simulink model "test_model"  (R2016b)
settings: Solver=VariableStepAuto  StartTime=0.0  StopTime=runtime  RelTol=1e-3
InitFcn:
  | clear mex
  | delete test_model_sfun.mexw64
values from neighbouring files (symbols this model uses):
  delta_T = 4 * [ 0,  0,  2.351e-4 ]    [modelParameters.m]
  Delta_T = cell(1,4)    [modelParameters.m]
  F_D = 1*randn(3,1)    [modelParameters.m]
  g = 9.81    [modelParameters.m]    (also in analyzeIMU_data.m = 9.8; getMomentOfInertia.m = 9.80665)
  Gamma_H = cell(1,4)    [modelParameters.m]
  have_motor_transient = 1    [modelParameters.m]
  height_controlled_o = (((Rm*If        + (((omega0_o * 2 * Rm * Kv * Kq      * Kd + 1)^2) - 1)/(4* Rm*Kv^2*Kq      * Kd))/Vb)*(Pmax - Pmin) + Pmin)    [modelParameters.m]
  i_0 = cell(1,4)    [modelParameters.m]
  If = 0.3836    [modelParameters.m]    (also in thrustDragConstantCalculations.m = [If0; If1; If2; If3]; Kd_error.m = I_0 * sign(rotor_speed_0) + I_1 * rotor_speed_0 + I_2 * roto)
  J = diag([ 0.0130 0.0140 0.0285 ])    [modelParameters.m]    (also in J_calc_bifilar.m = (16*pi^2*L./(m*g.*D.^2))\(t./n).^2)
  J_L = m_L/12*diag([y_L^2+z_L^2,x_L^2+z_L^2,x_L^2+y_L^2])    [modelParameters.m]
  J_r = cell(1,4)    [modelParameters.m]
  Jreq = 4.2012e-05    [modelParameters.m]
  Jxx = 0.0130    (= 0.013)    [modelParameters.m]
  Jyy = 0.0140    (= 0.014)    [modelParameters.m]
  Jzz = 0.0285    [modelParameters.m]
  K_d = cell(1,4)    [modelParameters.m]
  K_E = cell(1,4)    [modelParameters.m]
  K_H = cell(1,4)    [modelParameters.m]
  K_Q = cell(1,4)    [modelParameters.m]
  K_T = cell(1,4)    [modelParameters.m]
  K_V = cell(1,4)    [modelParameters.m]
  Kd = 1.4852e-07    [modelParameters.m]    (also in calcDragConstant.m = ((A'*A)^-1)*A'*b; thrustDragConstantCalculations.m = calcDragConstant(data, Pmin, Pmax, Rm, Kv, Kq, If); Kd_error.m = 1.0317e-07)
  Kh = 3.4574e-04    (= 0.00034574)    [modelParameters.m]
  Ki_mahony = 0.001    [modelParameters.m]
  Kp_mahony = 0.4    [modelParameters.m]
  Kq = 96.3422    [modelParameters.m]    (also in thrustDragConstantCalculations.m; Kd_error.m)
  Kt = 1.2007e-05    [modelParameters.m]    (also in calcThrustConstant.m = ((A'*A)^(-1))*(A'*T); thrustDragConstantCalculations.m = calcThrustConstant(data))
  Kv = 96.3422    [modelParameters.m]    (also in thrustDragConstantCalculations.m; Kd_error.m)
  m = 1.216    [modelParameters.m]
  m_L = 0    [modelParameters.m]
  omega0_o = sqrt((m*g)/(4*Kt))    [modelParameters.m]
  omega1_o = sqrt((m*g)/(4*Kt))    [modelParameters.m]
  omega2_o = sqrt((m*g)/(4*Kt))    [modelParameters.m]
  omega3_o = sqrt((m*g)/(4*Kt))    [modelParameters.m]
  omega_0 = cell(1,4)    [modelParameters.m]
  p0 = 0    [modelParameters.m]
  p_0 = cell(1,4)    [modelParameters.m]
  p_max = cell(1,4)    [modelParameters.m]
  phi0 = 0    [modelParameters.m]
  pitch_o = 0    [modelParameters.m]
  pitchrate_o = 0    [modelParameters.m]
  Pmax = 1    [modelParameters.m]    (also in thrustDragConstantCalculations.m = 200000; Kd_error.m = 200000)
  Pmin = 0    [modelParameters.m]    (also in thrustDragConstantCalculations.m = 100000; Kd_error.m = 100000)
  psi0 = 0    [modelParameters.m]
  q0 = 0    [modelParameters.m]
  Q_D = 0.05*randn(3,1)    [modelParameters.m]
  r0 = 0    [modelParameters.m]
  R_m = cell(1,4)    [modelParameters.m]
  r_oc = [ 0 ; 0 ; 0 ]    [modelParameters.m]
  r_oL = [0; 0; 0]    [modelParameters.m]
  rhx = 0.16    [modelParameters.m]
  rhy = 0.16    [modelParameters.m]
  rhz = 0.03    [modelParameters.m]
  Rm = 0.235    [modelParameters.m]    (also in thrustDragConstantCalculations.m = 0.2308; Kd_error.m = 0.2308)
  roll_o = 0    [modelParameters.m]
  rollrate_o = 0    [modelParameters.m]
  Tc = 0.04    [modelParameters.m]
  theta0 = 0    [modelParameters.m]
  Tq = 0.005    [modelParameters.m]
  u0 = 0    [modelParameters.m]
  v0 = 0    [modelParameters.m]
  Vb = 12.3    [modelParameters.m]    (also in calcDragConstant.m = [data.(6); data.(6); data.(6); data.(6)]; Kd_error.m = data.(6))
  w0 = 0    [modelParameters.m]
  x0 = 0    [modelParameters.m]
  x_controlled_o = 0    [modelParameters.m]
  x_o = 0    [modelParameters.m]
  x_vel_o = 0    [modelParameters.m]
  y0 = 0    [modelParameters.m]
  y_controlled_o = 0    [modelParameters.m]
  y_o = 0    [modelParameters.m]
  y_vel_o = 0    [modelParameters.m]
  yaw_controlled_o = 0    [modelParameters.m]
  yaw_o = 0    [modelParameters.m]
  yawrate_o = 0    [modelParameters.m]
  z0 = 0    [modelParameters.m]
  z_o = 0    [modelParameters.m]
  z_vel_o = 0    [modelParameters.m]
undefined symbols (not defined in the file or in its folder): Gamma_Omega, Gamma_T, Ki, Kp, r_h, slope, start, Ts, X0
libraries: simulink x32, Derivative x26, dsparch4 x6, vrlib x4
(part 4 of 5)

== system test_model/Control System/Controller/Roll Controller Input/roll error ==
  From Workspace1 : FromWorkspace  VariableName=roll_angle  SampleTime=Tq  Interpolate=off  OutputAfterFinalValue=Holding final value
  From Workspace4 : FromWorkspace  VariableName=roll_error  SampleTime=Tq  Interpolate=off  OutputAfterFinalValue=Holding final value
  roll_error : Outport
  roll_angle : Outport  Port=2
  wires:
  From Workspace4/1 -> roll_error/1
  From Workspace1/1 -> roll_angle/1

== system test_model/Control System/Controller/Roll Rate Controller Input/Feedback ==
  rollrate_error_model : Inport
  rollrate_model : Inport  Port=2
  rollrate_error : Outport
  rollrate : Outport  Port=2
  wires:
  rollrate_error_model/1 -> rollrate_error/1
  rollrate_model/1 -> rollrate/1

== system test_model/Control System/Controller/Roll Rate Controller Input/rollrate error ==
  From Workspace1 : FromWorkspace  VariableName=rollrate  SampleTime=Tq  Interpolate=off  OutputAfterFinalValue=Holding final value
  From Workspace5 : FromWorkspace  VariableName=rollrate_error  SampleTime=Tq  Interpolate=off  OutputAfterFinalValue=Holding final value
  rollrate_error : Outport
  rollrate : Outport  Port=2
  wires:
  From Workspace5/1 -> rollrate_error/1
  From Workspace1/1 -> rollrate/1

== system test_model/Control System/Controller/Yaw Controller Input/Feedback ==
  yaw_error_model : Inport
  yaw_angle_model : Inport  Port=2
  yaw_error : Outport
  yaw_angle : Outport  Port=2
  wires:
  yaw_error_model/1 -> yaw_error/1
  yaw_angle_model/1 -> yaw_angle/1

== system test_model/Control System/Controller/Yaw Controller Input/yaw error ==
  From Workspace1 : FromWorkspace  VariableName=yaw_angle  SampleTime=Tc  Interpolate=off  OutputAfterFinalValue=Holding final value
  From Workspace7 : FromWorkspace  VariableName=yaw_error  SampleTime=Tc  Interpolate=off  OutputAfterFinalValue=Holding final value
  yaw_error : Outport
  yaw_angle : Outport  Port=2
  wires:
  From Workspace7/1 -> yaw_error/1
  From Workspace1/1 -> yaw_angle/1

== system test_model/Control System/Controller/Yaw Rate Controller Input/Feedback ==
  yawrate_error_model : Inport
  yawrate_model : Inport  Port=2
  yawrate_error : Outport
  yawrate : Outport  Port=2
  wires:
  yawrate_error_model/1 -> yawrate_error/1
  yawrate_model/1 -> yawrate/1

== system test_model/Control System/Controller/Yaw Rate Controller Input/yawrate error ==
  From Workspace1 : FromWorkspace  VariableName=yawrate  SampleTime=Tq  Interpolate=off  OutputAfterFinalValue=Holding final value
  From Workspace8 : FromWorkspace  VariableName=yawrate_error  SampleTime=Tq  Interpolate=off  OutputAfterFinalValue=Holding final value
  yawrate_error : Outport
  yawrate : Outport  Port=2
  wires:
  From Workspace8/1 -> yawrate_error/1
  From Workspace1/1 -> yawrate/1

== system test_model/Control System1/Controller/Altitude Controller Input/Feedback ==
  z_error_model : Inport
  z_position_model : Inport  Port=2
  z_error : Outport
  z_position : Outport  Port=2
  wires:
  z_error_model/1 -> z_error/1
  z_position_model/1 -> z_position/1

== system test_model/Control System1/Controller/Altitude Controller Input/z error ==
  From Workspace1 : FromWorkspace  VariableName=z_position  SampleTime=Tc  Interpolate=off  OutputAfterFinalValue=Holding final value
  From Workspace6 : FromWorkspace  VariableName=z_error  SampleTime=Tc  Interpolate=off  OutputAfterFinalValue=Holding final value
  z_error : Outport
  z_position : Outport  Port=2
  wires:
  From Workspace6/1 -> z_error/1
  From Workspace1/1 -> z_position/1

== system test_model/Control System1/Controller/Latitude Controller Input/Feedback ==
  x_error_model : Inport
  x_position_model : Inport  Port=2
  x_error : Outport
  x_position : Outport  Port=2
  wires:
  x_error_model/1 -> x_error/1
  x_position_model/1 -> x_position/1

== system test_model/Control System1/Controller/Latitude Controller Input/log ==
  From Workspace : FromWorkspace  VariableName=x_error  SampleTime=Tc  Interpolate=off  OutputAfterFinalValue=Holding final value
  From Workspace1 : FromWorkspace  VariableName=x_position  SampleTime=Tc  Interpolate=off  OutputAfterFinalValue=Holding final value
  x_error : Outport
  x_position : Outport  Port=2
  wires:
  From Workspace/1 -> x_error/1
  From Workspace1/1 -> x_position/1

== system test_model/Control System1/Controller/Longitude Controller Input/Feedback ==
  y_error_model : Inport
  y_position_model : Inport  Port=2
  y_error : Outport
  y_position : Outport  Port=2
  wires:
  y_error_model/1 -> y_error/1
  y_position_model/1 -> y_position/1

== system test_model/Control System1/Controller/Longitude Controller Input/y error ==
  From Workspace1 : FromWorkspace  VariableName=y_position  SampleTime=Tc  Interpolate=off  OutputAfterFinalValue=Holding final value
  From Workspace3 : FromWorkspace  VariableName=y_error  SampleTime=Tc  Interpolate=off  OutputAfterFinalValue=Holding final value
  y_error : Outport
  y_position : Outport  Port=2
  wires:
  From Workspace3/1 -> y_error/1
  From Workspace1/1 -> y_position/1

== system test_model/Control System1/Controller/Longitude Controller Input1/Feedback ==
  y_vel_error_model : Inport
  y_vel_model : Inport  Port=2
  y_vel_error : Outport
  y_vel : Outport  Port=2
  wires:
  y_vel_error_model/1 -> y_vel_error/1
  y_vel_model/1 -> y_vel/1

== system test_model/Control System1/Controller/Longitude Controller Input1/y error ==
  From Workspace1 : FromWorkspace  VariableName=y_vel  SampleTime=Tc  Interpolate=off  OutputAfterFinalValue=Holding final value
  From Workspace3 : FromWorkspace  VariableName=y_vel_error  SampleTime=Tc  Interpolate=off  OutputAfterFinalValue=Holding final value
  y_vel_error : Outport
  y_vel : Outport  Port=2
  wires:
  From Workspace3/1 -> y_vel_error/1
  From Workspace1/1 -> y_vel/1

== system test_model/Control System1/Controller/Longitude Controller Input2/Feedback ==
  x_vel_error_model : Inport
  x_vel_model : Inport  Port=2
  x_vel_error : Outport
  x_vel : Outport  Port=2
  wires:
  x_vel_error_model/1 -> x_vel_error/1
  x_vel_model/1 -> x_vel/1

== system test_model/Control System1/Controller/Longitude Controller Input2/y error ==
  From Workspace1 : FromWorkspace  VariableName=x_vel  SampleTime=Tc  Interpolate=off  OutputAfterFinalValue=Holding final value
  From Workspace3 : FromWorkspace  VariableName=x_vel_error  SampleTime=Tc  Interpolate=off  OutputAfterFinalValue=Holding final value
  x_vel_error : Outport
  x_vel : Outport  Port=2
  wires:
  From Workspace3/1 -> x_vel_error/1
  From Workspace1/1 -> x_vel/1

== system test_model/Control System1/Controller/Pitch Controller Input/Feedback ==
  pitch_error_model : Inport
  pitch_angle_model : Inport  Port=2
  pitch_error : Outport
  pitch_angle : Outport  Port=2
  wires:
  pitch_error_model/1 -> pitch_error/1
  pitch_angle_model/1 -> pitch_angle/1

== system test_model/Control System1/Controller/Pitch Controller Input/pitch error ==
  From Workspace : FromWorkspace  VariableName=pitch_error  SampleTime=Tq  Interpolate=off  OutputAfterFinalValue=Holding final value
  From Workspace1 : FromWorkspace  VariableName=pitch_angle  SampleTime=Tq  Interpolate=off  OutputAfterFinalValue=Holding final value
  pitch_error : Outport
  pitch_angle : Outport  Port=2
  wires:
  From Workspace/1 -> pitch_error/1
  From Workspace1/1 -> pitch_angle/1

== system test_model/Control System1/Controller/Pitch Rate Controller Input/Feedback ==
  pitchrate_error_model : Inport
  pitchrate_model : Inport  Port=2
  pitchrate_error : Outport
  pitchrate : Outport  Port=2
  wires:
  pitchrate_error_model/1 -> pitchrate_error/1
  pitchrate_model/1 -> pitchrate/1

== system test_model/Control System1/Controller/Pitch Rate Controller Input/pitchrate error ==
  From Workspace1 : FromWorkspace  VariableName=pitchrate  SampleTime=Tq  Interpolate=off  OutputAfterFinalValue=Holding final value
  From Workspace2 : FromWorkspace  VariableName=pitchrate_error  SampleTime=Tq  Interpolate=off  OutputAfterFinalValue=Holding final value
  pitchrate_error : Outport
  pitchrate : Outport  Port=2
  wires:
  From Workspace2/1 -> pitchrate_error/1
  From Workspace1/1 -> pitchrate/1

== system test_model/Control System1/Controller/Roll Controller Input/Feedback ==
  roll_error_model : Inport
  roll_angle_model : Inport  Port=2
  roll_error : Outport
  roll_angle : Outport  Port=2
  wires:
  roll_error_model/1 -> roll_error/1
  roll_angle_model/1 -> roll_angle/1

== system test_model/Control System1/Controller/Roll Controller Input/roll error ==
  From Workspace1 : FromWorkspace  VariableName=roll_angle  SampleTime=Tq  Interpolate=off  OutputAfterFinalValue=Holding final value
  From Workspace4 : FromWorkspace  VariableName=roll_error  SampleTime=Tq  Interpolate=off  OutputAfterFinalValue=Holding final value
  roll_error : Outport
  roll_angle : Outport  Port=2
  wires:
  From Workspace4/1 -> roll_error/1
  From Workspace1/1 -> roll_angle/1

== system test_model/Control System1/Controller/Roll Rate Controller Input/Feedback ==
  rollrate_error_model : Inport
  rollrate_model : Inport  Port=2
  rollrate_error : Outport
  rollrate : Outport  Port=2
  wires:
  rollrate_error_model/1 -> rollrate_error/1
  rollrate_model/1 -> rollrate/1

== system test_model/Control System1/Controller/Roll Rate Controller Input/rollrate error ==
  From Workspace1 : FromWorkspace  VariableName=rollrate  SampleTime=Tq  Interpolate=off  OutputAfterFinalValue=Holding final value
  From Workspace5 : FromWorkspace  VariableName=rollrate_error  SampleTime=Tq  Interpolate=off  OutputAfterFinalValue=Holding final value
  rollrate_error : Outport
  rollrate : Outport  Port=2
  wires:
  From Workspace5/1 -> rollrate_error/1
  From Workspace1/1 -> rollrate/1

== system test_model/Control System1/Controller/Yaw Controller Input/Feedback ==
  yaw_error_model : Inport
  yaw_angle_model : Inport  Port=2
  yaw_error : Outport
  yaw_angle : Outport  Port=2
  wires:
  yaw_error_model/1 -> yaw_error/1
  yaw_angle_model/1 -> yaw_angle/1

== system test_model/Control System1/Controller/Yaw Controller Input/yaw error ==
  From Workspace1 : FromWorkspace  VariableName=yaw_angle  SampleTime=Tc  Interpolate=off  OutputAfterFinalValue=Holding final value
  From Workspace7 : FromWorkspace  VariableName=yaw_error  SampleTime=Tc  Interpolate=off  OutputAfterFinalValue=Holding final value
  yaw_error : Outport
  yaw_angle : Outport  Port=2
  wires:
  From Workspace7/1 -> yaw_error/1
  From Workspace1/1 -> yaw_angle/1

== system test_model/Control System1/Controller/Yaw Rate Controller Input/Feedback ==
  yawrate_error_model : Inport
  yawrate_model : Inport  Port=2
  yawrate_error : Outport
  yawrate : Outport  Port=2
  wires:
  yawrate_error_model/1 -> yawrate_error/1
  yawrate_model/1 -> yawrate/1

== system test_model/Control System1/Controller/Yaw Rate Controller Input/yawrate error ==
  From Workspace1 : FromWorkspace  VariableName=yawrate  SampleTime=Tq  Interpolate=off  OutputAfterFinalValue=Holding final value
  From Workspace8 : FromWorkspace  VariableName=yawrate_error  SampleTime=Tq  Interpolate=off  OutputAfterFinalValue=Holding final value
  yawrate_error : Outport
  yawrate : Outport  Port=2
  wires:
  From Workspace8/1 -> yawrate_error/1
  From Workspace1/1 -> yawrate/1

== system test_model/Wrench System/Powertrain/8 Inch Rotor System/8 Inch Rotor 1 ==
  alpha : Inport
  omega : Inport  Port=2
  v : Inport  Port=3
  Omega : Inport  Port=4
  8 Inch Rotor : MATLAB Function
  Delta_T : Constant  Value=Delta_T
  Gamma_H : Constant  Value=Gamma_H
  Gamma_Omega : Constant  Value=Gamma_Omega
  Gamma_T : Constant  Value=Gamma_T
  J_r : Constant  Value=J_r
  K_H : Constant  Value=K_H
  K_T : Constant  Value=K_T
  K_d : Constant  Value=K_d
  Scope : Scope
  r_h : Constant  Value=r_h
  F : Outport
  Q : Outport  Port=2
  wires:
  8 Inch Rotor/2(Q) -> Q/1
  8 Inch Rotor/1(F) -> Scope/1, F/1
  Omega/1 -> 8 Inch Rotor/4(Omega)
  v/1 -> 8 Inch Rotor/3(v)
  K_T/1 -> 8 Inch Rotor/5(K_T)
  Gamma_Omega/1 -> 8 Inch Rotor/12(Gamma_Omega)
  Gamma_H/1 -> 8 Inch Rotor/11(Gamma_H)
  Gamma_T/1 -> 8 Inch Rotor/10(Gamma_T)
  Delta_T/1 -> 8 Inch Rotor/9(Delta_T)
  r_h/1 -> 8 Inch Rotor/8(r_h)
  K_d/1 -> 8 Inch Rotor/7(K_d)
  K_H/1 -> 8 Inch Rotor/6(K_H)
  omega/1 -> 8 Inch Rotor/1(omega)
  alpha/1 -> 8 Inch Rotor/2(alpha)
  J_r/1 -> 8 Inch Rotor/13(J_r)

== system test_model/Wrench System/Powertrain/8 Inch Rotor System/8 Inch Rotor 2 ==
  alpha : Inport
  omega : Inport  Port=2
  v : Inport  Port=3
  Omega : Inport  Port=4
  8 Inch Rotor : MATLAB Function
  Delta_T : Constant  Value=Delta_T
  Gamma_H : Constant  Value=Gamma_H
  Gamma_Omega : Constant  Value=Gamma_Omega
  Gamma_T : Constant  Value=Gamma_T
  J_r : Constant  Value=J_r
  K_H : Constant  Value=K_H
  K_T : Constant  Value=K_T
  K_d : Constant  Value=K_d
  r_h : Constant  Value=r_h
  F : Outport
  Q : Outport  Port=2
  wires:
  8 Inch Rotor/2(Q) -> Q/1
  8 Inch Rotor/1(F) -> F/1
  Omega/1 -> 8 Inch Rotor/4(Omega)
  v/1 -> 8 Inch Rotor/3(v)
  K_T/1 -> 8 Inch Rotor/5(K_T)
  Gamma_Omega/1 -> 8 Inch Rotor/12(Gamma_Omega)
  Gamma_H/1 -> 8 Inch Rotor/11(Gamma_H)
  Gamma_T/1 -> 8 Inch Rotor/10(Gamma_T)
  Delta_T/1 -> 8 Inch Rotor/9(Delta_T)
  r_h/1 -> 8 Inch Rotor/8(r_h)
  K_d/1 -> 8 Inch Rotor/7(K_d)
  K_H/1 -> 8 Inch Rotor/6(K_H)
  omega/1 -> 8 Inch Rotor/1(omega)
  alpha/1 -> 8 Inch Rotor/2(alpha)
  J_r/1 -> 8 Inch Rotor/13(J_r)

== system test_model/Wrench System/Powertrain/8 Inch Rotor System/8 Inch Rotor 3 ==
  alpha : Inport
  omega : Inport  Port=2
  v : Inport  Port=3
  Omega : Inport  Port=4
  8 Inch Rotor : MATLAB Function
  Delta_T : Constant  Value=Delta_T
  Gamma_H : Constant  Value=Gamma_H
  Gamma_Omega : Constant  Value=Gamma_Omega
  Gamma_T : Constant  Value=Gamma_T
  J_r : Constant  Value=J_r
  K_H : Constant  Value=K_H
  K_T : Constant  Value=K_T
  K_d : Constant  Value=K_d
  r_h : Constant  Value=r_h
  F : Outport
  Q : Outport  Port=2
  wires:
  8 Inch Rotor/2(Q) -> Q/1
  8 Inch Rotor/1(F) -> F/1
  Omega/1 -> 8 Inch Rotor/4(Omega)
  v/1 -> 8 Inch Rotor/3(v)
  K_T/1 -> 8 Inch Rotor/5(K_T)
  Gamma_Omega/1 -> 8 Inch Rotor/12(Gamma_Omega)
  Gamma_H/1 -> 8 Inch Rotor/11(Gamma_H)
  Gamma_T/1 -> 8 Inch Rotor/10(Gamma_T)
  Delta_T/1 -> 8 Inch Rotor/9(Delta_T)
  r_h/1 -> 8 Inch Rotor/8(r_h)
  K_d/1 -> 8 Inch Rotor/7(K_d)
  K_H/1 -> 8 Inch Rotor/6(K_H)
  omega/1 -> 8 Inch Rotor/1(omega)
  alpha/1 -> 8 Inch Rotor/2(alpha)
  J_r/1 -> 8 Inch Rotor/13(J_r)

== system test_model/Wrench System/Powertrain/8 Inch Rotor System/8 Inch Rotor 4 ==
  alpha : Inport
  omega : Inport  Port=2
  v : Inport  Port=3
  Omega : Inport  Port=4
  8 Inch Rotor : MATLAB Function
  Delta_T : Constant  Value=Delta_T
  Gamma_H : Constant  Value=Gamma_H
  Gamma_Omega : Constant  Value=Gamma_Omega
  Gamma_T : Constant  Value=Gamma_T
  J_r : Constant  Value=J_r
  K_H : Constant  Value=K_H
  K_T : Constant  Value=K_T
  K_d : Constant  Value=K_d
  r_h : Constant  Value=r_h
  F : Outport
  Q : Outport  Port=2
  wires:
  8 Inch Rotor/2(Q) -> Q/1
  8 Inch Rotor/1(F) -> F/1
  Omega/1 -> 8 Inch Rotor/4(Omega)
  v/1 -> 8 Inch Rotor/3(v)
  K_T/1 -> 8 Inch Rotor/5(K_T)
  Gamma_Omega/1 -> 8 Inch Rotor/12(Gamma_Omega)
  Gamma_H/1 -> 8 Inch Rotor/11(Gamma_H)
  Gamma_T/1 -> 8 Inch Rotor/10(Gamma_T)
  Delta_T/1 -> 8 Inch Rotor/9(Delta_T)
  r_h/1 -> 8 Inch Rotor/8(r_h)
  K_d/1 -> 8 Inch Rotor/7(K_d)
  K_H/1 -> 8 Inch Rotor/6(K_H)
  omega/1 -> 8 Inch Rotor/1(omega)
  alpha/1 -> 8 Inch Rotor/2(alpha)
  J_r/1 -> 8 Inch Rotor/13(J_r)

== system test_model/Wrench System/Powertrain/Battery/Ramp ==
  Clock : Clock
  Constant : Constant  DisableCoverage=on  Value=start  OutDataTypeStr=Inherit: Inherit via back propagation
  Constant1 : Constant  DisableCoverage=on  Value=X0  OutDataTypeStr=Inherit: Inherit via back propagation
  Output : Sum  Inputs=|++
  Product : Product  DisableCoverage=on
  Step : Step  DisableCoverage=on  Time=start  After=slope  SampleTime=0
  Sum : Sum  DisableCoverage=on  Inputs=|+-
  Out1 : Outport
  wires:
  Clock/1 -> Sum/1
  Constant/1 -> Sum/2
  Sum/1 -> Product/2
  Output/1 -> Out1/1
  Constant1/1 -> Output/2
  Product/1 -> Output/1
  Step/1 -> Product/1

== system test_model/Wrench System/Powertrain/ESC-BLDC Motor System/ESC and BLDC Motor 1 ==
  p : Inport
  V_b : Inport  Port=2
  "BLDC Motor " : MATLAB Function  TreatAsAtomicUnit=on
  BLDC Motor (no transient) : MATLAB Function  TreatAsAtomicUnit=on
  "ESC " : MATLAB Function  TreatAsAtomicUnit=on
  Integrator : Integrator  InitialCondition=omega_0  ContinuousStateAttributes='omega'
  J_r : Constant  Value=J_r
  K_E : Constant  Value=K_E
  K_Q : Constant  Value=K_Q
  K_V : Constant  Value=K_V
  K_d : Constant  Value=K_d
  R_m : Constant  Value=R_m
  alpha_switch : Switch  Criteria=u2 ~= 0
  i_0 : Constant  Value=i_0
  motor_transient_choice : Constant  Value=have_motor_transient
  omega_switch : Switch  Criteria=u2 ~= 0
  p_0 : Constant  Value=p_0
  p_max : Constant  Value=p_max
  alpha : Outport
  omega : Outport  Port=2
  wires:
  motor_transient_choice/1 -> omega_switch/2, alpha_switch/2
  omega_switch/1 -> omega/1
  alpha_switch/1 -> alpha/1
  BLDC Motor (no transient)/2(omega) -> omega_switch/3
  BLDC Motor (no transient)/1(alpha) -> alpha_switch/3
  Integrator/1 -> omega_switch/1, "BLDC Motor "/2(omega)
  "ESC "/1(V) -> BLDC Motor (no transient)/1(V), "BLDC Motor "/1(V)
  p/1 -> "ESC "/1(p)
  V_b/1 -> "ESC "/2(V_b)
  K_E/1 -> "ESC "/3(K_E)
  p_0/1 -> "ESC "/4(p_0)
  p_max/1 -> "ESC "/5(p_max)
  J_r/1 -> "BLDC Motor "/8(J_r)
  R_m/1 -> BLDC Motor (no transient)/2(R_m), "BLDC Motor "/3(R_m)
  "BLDC Motor "/1(alpha) -> alpha_switch/1, Integrator/1
  K_Q/1 -> BLDC Motor (no transient)/3(K_Q), "BLDC Motor "/4(K_Q)
  K_V/1 -> BLDC Motor (no transient)/4(K_V), "BLDC Motor "/5(K_V)
  i_0/1 -> BLDC Motor (no transient)/5(i_0), "BLDC Motor "/6(i_0)
  K_d/1 -> BLDC Motor (no transient)/6(K_d), "BLDC Motor "/7(K_d)

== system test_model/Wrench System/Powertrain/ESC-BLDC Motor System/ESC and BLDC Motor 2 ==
  p : Inport
  V_b : Inport  Port=2
  "BLDC Motor " : MATLAB Function  TreatAsAtomicUnit=on
  BLDC Motor (no transient) : MATLAB Function  TreatAsAtomicUnit=on
  "ESC " : MATLAB Function  TreatAsAtomicUnit=on
  Integrator : Integrator  InitialCondition=omega_0  ContinuousStateAttributes='omega'
  J_r : Constant  Value=J_r
  K_E : Constant  Value=K_E
  K_Q : Constant  Value=K_Q
  K_V : Constant  Value=K_V
  K_d : Constant  Value=K_d
  R_m : Constant  Value=R_m
  alpha_switch : Switch  Criteria=u2 ~= 0
  i_0 : Constant  Value=i_0
  motor_transient_choice : Constant  Value=have_motor_transient
  omega_switch : Switch  Criteria=u2 ~= 0
  p_0 : Constant  Value=p_0
  p_max : Constant  Value=p_max
  alpha : Outport
  omega : Outport  Port=2
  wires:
  motor_transient_choice/1 -> omega_switch/2, alpha_switch/2
  omega_switch/1 -> omega/1
  alpha_switch/1 -> alpha/1
  BLDC Motor (no transient)/2(omega) -> omega_switch/3
  BLDC Motor (no transient)/1(alpha) -> alpha_switch/3
  Integrator/1 -> omega_switch/1, "BLDC Motor "/2(omega)
  "ESC "/1(V) -> BLDC Motor (no transient)/1(V), "BLDC Motor "/1(V)
  p/1 -> "ESC "/1(p)
  V_b/1 -> "ESC "/2(V_b)
  K_E/1 -> "ESC "/3(K_E)
  p_0/1 -> "ESC "/4(p_0)
  p_max/1 -> "ESC "/5(p_max)
  J_r/1 -> "BLDC Motor "/8(J_r)
  R_m/1 -> BLDC Motor (no transient)/2(R_m), "BLDC Motor "/3(R_m)
  "BLDC Motor "/1(alpha) -> alpha_switch/1, Integrator/1
  K_Q/1 -> BLDC Motor (no transient)/3(K_Q), "BLDC Motor "/4(K_Q)
  K_V/1 -> BLDC Motor (no transient)/4(K_V), "BLDC Motor "/5(K_V)
  i_0/1 -> BLDC Motor (no transient)/5(i_0), "BLDC Motor "/6(i_0)
  K_d/1 -> BLDC Motor (no transient)/6(K_d), "BLDC Motor "/7(K_d)

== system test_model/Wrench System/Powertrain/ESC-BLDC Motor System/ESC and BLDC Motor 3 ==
  p : Inport
  V_b : Inport  Port=2
  "BLDC Motor " : MATLAB Function  TreatAsAtomicUnit=on
  BLDC Motor (no transient) : MATLAB Function  TreatAsAtomicUnit=on
  "ESC " : MATLAB Function  TreatAsAtomicUnit=on
  Integrator : Integrator  InitialCondition=omega_0  ContinuousStateAttributes='omega'
  J_r : Constant  Value=J_r
  K_E : Constant  Value=K_E
  K_Q : Constant  Value=K_Q
  K_V : Constant  Value=K_V
  K_d : Constant  Value=K_d
  R_m : Constant  Value=R_m
  alpha_switch : Switch  Criteria=u2 ~= 0
  i_0 : Constant  Value=i_0
  motor_transient_choice : Constant  Value=have_motor_transient
  omega_switch : Switch  Criteria=u2 ~= 0
  p_0 : Constant  Value=p_0
  p_max : Constant  Value=p_max
  alpha : Outport
  omega : Outport  Port=2
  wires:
  motor_transient_choice/1 -> omega_switch/2, alpha_switch/2
  omega_switch/1 -> omega/1
  alpha_switch/1 -> alpha/1
  BLDC Motor (no transient)/2(omega) -> omega_switch/3
  BLDC Motor (no transient)/1(alpha) -> alpha_switch/3
  Integrator/1 -> omega_switch/1, "BLDC Motor "/2(omega)
  "ESC "/1(V) -> BLDC Motor (no transient)/1(V), "BLDC Motor "/1(V)
  p/1 -> "ESC "/1(p)
  V_b/1 -> "ESC "/2(V_b)
  K_E/1 -> "ESC "/3(K_E)
  p_0/1 -> "ESC "/4(p_0)
  p_max/1 -> "ESC "/5(p_max)
  J_r/1 -> "BLDC Motor "/8(J_r)
  R_m/1 -> BLDC Motor (no transient)/2(R_m), "BLDC Motor "/3(R_m)
  "BLDC Motor "/1(alpha) -> alpha_switch/1, Integrator/1
  K_Q/1 -> BLDC Motor (no transient)/3(K_Q), "BLDC Motor "/4(K_Q)
  K_V/1 -> BLDC Motor (no transient)/4(K_V), "BLDC Motor "/5(K_V)
  i_0/1 -> BLDC Motor (no transient)/5(i_0), "BLDC Motor "/6(i_0)
  K_d/1 -> BLDC Motor (no transient)/6(K_d), "BLDC Motor "/7(K_d)

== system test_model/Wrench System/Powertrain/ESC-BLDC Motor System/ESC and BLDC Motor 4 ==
  p : Inport
  V_b : Inport  Port=2
  "BLDC Motor " : MATLAB Function  TreatAsAtomicUnit=on
  BLDC Motor (no transient) : MATLAB Function  TreatAsAtomicUnit=on
  "ESC " : MATLAB Function  TreatAsAtomicUnit=on
  Integrator : Integrator  InitialCondition=omega_0  ContinuousStateAttributes='omega'
  J_r : Constant  Value=J_r
  K_E : Constant  Value=K_E
  K_Q : Constant  Value=K_Q
  K_V : Constant  Value=K_V
  K_d : Constant  Value=K_d
  R_m : Constant  Value=R_m
  alpha_switch : Switch  Criteria=u2 ~= 0
  i_0 : Constant  Value=i_0
  motor_transient_choice : Constant  Value=have_motor_transient
  omega_switch : Switch  Criteria=u2 ~= 0
  p_0 : Constant  Value=p_0
  p_max : Constant  Value=p_max
  alpha : Outport
  omega : Outport  Port=2
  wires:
  motor_transient_choice/1 -> omega_switch/2, alpha_switch/2
  omega_switch/1 -> omega/1
  alpha_switch/1 -> alpha/1
  BLDC Motor (no transient)/2(omega) -> omega_switch/3
  BLDC Motor (no transient)/1(alpha) -> alpha_switch/3
  Integrator/1 -> omega_switch/1, "BLDC Motor "/2(omega)
  "ESC "/1(V) -> BLDC Motor (no transient)/1(V), "BLDC Motor "/1(V)
  p/1 -> "ESC "/1(p)
  V_b/1 -> "ESC "/2(V_b)
  K_E/1 -> "ESC "/3(K_E)
  p_0/1 -> "ESC "/4(p_0)
  p_max/1 -> "ESC "/5(p_max)
  J_r/1 -> "BLDC Motor "/8(J_r)
  R_m/1 -> BLDC Motor (no transient)/2(R_m), "BLDC Motor "/3(R_m)
  "BLDC Motor "/1(alpha) -> alpha_switch/1, Integrator/1
  K_Q/1 -> BLDC Motor (no transient)/3(K_Q), "BLDC Motor "/4(K_Q)
  K_V/1 -> BLDC Motor (no transient)/4(K_V), "BLDC Motor "/5(K_V)
  i_0/1 -> BLDC Motor (no transient)/5(i_0), "BLDC Motor "/6(i_0)
  K_d/1 -> BLDC Motor (no transient)/6(K_d), "BLDC Motor "/7(K_d)

== matlab function test_model/Actuation/Gravity

 ==
function E_Fg = gravity(m, g)

E_Fg = [0; 0; m*g];

== matlab function test_model/Actuation/Lbe





 ==
function E_ro  = linear_body_earth_conversion(B_vo, euler_angles)

euler_rates = zeros(3,1);
E_ro = zeros(3,1);

phi = euler_angles(1);
theta = euler_angles(2);
psi = euler_angles(3);

Leb = [cos(theta)*cos(psi), sin(phi)*sin(theta)*cos(psi)-cos(phi)*sin(psi), cos(phi)*sin(theta)*cos(psi)+sin(phi)*sin(psi); ...
       cos(theta)*sin(psi), sin(phi)*sin(theta)*sin(psi)+cos(phi)*cos(psi), cos(phi)*sin(theta)*sin(psi)-sin(phi)*cos(psi); ...
           -sin(theta)    ,                sin(phi)*cos(theta)            ,                 cos(phi)*cos(theta)           ];

E_ro = Leb * B_vo;

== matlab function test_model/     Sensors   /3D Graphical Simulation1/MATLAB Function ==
function y = eigenaxis_ucart(u)


if abs(u(1))< 0.0001
    u(1) = 0.0001;
end

if abs(u(2))< 0.0001
    u(2) = 0.0001;
end

if abs(u(3))< 0.0001
    u(3) = 0.0001;
end

u = [ -u(1); -u(2); u(3) ];% [Pitch, Yaw, Roll] 

C11 = cos(u(2))*cos(u(3));
C12 = cos(u(2))*sin(u(3));
C13 = -sin(u(2));
C21 = sin(u(1))*sin(u(2))*cos(u(3))-cos(u(1))*sin(u(3));
C22 = sin(u(1))*sin(u(2))*sin(u(3))+cos(u(1))*cos(u(3));
C23 = sin(u(1))*cos(u(2));
C31 = cos(u(1))*sin(u(2))*cos(u(3))+sin(u(1))*sin(u(3));
C32 = cos(u(1))*sin(u(2))*sin(u(3))-sin(u(1))*cos(u(3));
C33 = cos(u(1))*cos(u(2));
    
theta = acos(0.5*(C11+C22+C33-1));

e = [C23-C32; C31-C13; C12-C21]/(2*sin(theta));
    
y = [e; theta];

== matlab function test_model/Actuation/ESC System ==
function Vb_eff   = ESC(P, Pmin, Pmax, Vb)

P1 = P(1);
P2 = P(2);
P3 = P(3);
P4 = P(4);

% Define u_Pi for each of the rotors, limiting it to be greater than 0
u_P0 = (P1 - Pmin) / (Pmax - Pmin);
u_P1 = (P2 - Pmin) / (Pmax - Pmin);
u_P2 = (P3 - Pmin) / (Pmax - Pmin);
u_P3 = (P4 - Pmin) / (Pmax - Pmin);


% Determine the effective battery voltage from each ESC
Vb_eff_0 = u_P0 * Vb;
Vb_eff_1 = u_P1 * Vb;
Vb_eff_2 = u_P2 * Vb;
Vb_eff_3 = u_P3 * Vb;
    
Vb_eff = [Vb_eff_0, Vb_eff_1, Vb_eff_2, Vb_eff_3];

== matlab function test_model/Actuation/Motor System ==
function w_dot = motor(Vb_eff, w, Rm, Kv, Kq, Kd, If, Jreq)

% Define each motors effective battery voltage
Vb_eff_0 = Vb_eff(1);
Vb_eff_1 = Vb_eff(2);
Vb_eff_2 = Vb_eff(3);
Vb_eff_3 = Vb_eff(4);

% Determine the angular velocity of each rotor from feedback
w_0 = w(1);
w_1 = w(2);
w_2 = w(3);
w_3 = w(4);

% Determine angular acceleration of each rotor
w_0_dot = 1/(Jreq*Rm*Kq) * Vb_eff_0 - 1/(Jreq*Rm*Kq*Kv) * w_0 - 1/(Jreq*Kq)*If - (Kd/Jreq) * w_0^2;
w_1_dot = 1/(Jreq*Rm*Kq) * Vb_eff_1 - 1/(Jreq*Rm*Kq*Kv) * w_1 - 1/(Jreq*Kq)*If - (Kd/Jreq) * w_1^2;
w_2_dot = 1/(Jreq*Rm*Kq) * Vb_eff_2 - 1/(Jreq*Rm*Kq*Kv) * w_2 - 1/(Jreq*Kq)*If - (Kd/Jreq) * w_2^2;
w_3_dot = 1/(Jreq*Rm*Kq) * Vb_eff_3 - 1/(Jreq*Rm*Kq*Kv) * w_3 - 1/(Jreq*Kq)*If - (Kd/Jreq) * w_3^2;

w_dot = [w_0_dot, w_1_dot, w_2_dot, w_3_dot];

== matlab function test_model/Actuation/Rotor System







 ==
function [B_omega_dot, B_vo_dot, B_F]= rotor(w_dot, w, B_Fg, B_omega, B_vo, m, Kt, Kd, rhx, rhy, rhz, Jreq, Jxx, Jyy, Jzz, r_oc, Kh, delta_T)

% Create J vector
J = [Jxx,  0 ,  0 ; ...
      0 , Jyy,  0 ; ...
      0 ,  0 , Jzz;];
  
r_oc_X = [0, -r_oc(3), r_oc(2); r_oc(3), 0, -r_oc(1); -r_oc(2), r_oc(1), 0];

% Create r_hi vector
rh_0 = [-rhx; rhy; -rhz];
rh_1 = [rhx; rhy; -rhz];
rh_2 = [-rhx; -rhy; -rhz];
rh_3 = [rhx; -rhy; -rhz];

% Calculate rotor hub velocity
vh_0 = B_vo + cross(B_omega,rh_0);
vh_1 = B_vo + cross(B_omega,rh_1); 
vh_2 = B_vo + cross(B_omega,rh_2); 
vh_3 = B_vo + cross(B_omega,rh_3); 

% Define 3x3 Identity Matrix
I = eye(3);

% Create gamma vectors
gamma_Ti = [0; 0; -1];
gamma_omega_03 = [0; 0; 1];  %Rotors 0 and 3 use this gamma_omega vector
gamma_omega_12 = [0; 0; -1]; %Rotors 1 and 2 use this gamma_omega vector
gamma_Hi = [ 1 0 0 ; 0 1 0 ; 0 0 0 ];

% Define angular velocities for each rotor
w_0 = w(1);
w_1 = w(2);
w_2 = w(3);
w_3 = w(4);

% Define angular acceleration for each rotor
w_0_dot = w_dot(1);
w_1_dot = w_dot(2);
w_2_dot = w_dot(3);
w_3_dot = w_dot(4);

% Define the thrust force
T_0 = (Kt * w_0 * w_0 + delta_T * vh_0 * w_0) * gamma_Ti; 
T_1 = (Kt * w_1 * w_1 + delta_T * vh_1 * w_1) * gamma_Ti;
T_2 = (Kt * w_2 * w_2 + delta_T * vh_2 * w_2) * gamma_Ti;
T_3 = (Kt * w_3 * w_3 + delta_T * vh_3 * w_3) * gamma_Ti;

% Define the in plane drag force
H_0 = -Kh * w_0 * gamma_Hi * vh_0;
H_1 = -Kh * w_1 * gamma_Hi * vh_1;
H_2 = -Kh * w_2 * gamma_Hi * vh_2;
H_3 = -Kh * w_3 * gamma_Hi * vh_3;

% Define the rotor force in the z-direction from each rotor
B_Fr_0 = T_0 + H_0;
B_Fr_1 = T_1 + H_1;
B_Fr_2 = T_2 + H_2;
B_Fr_3 = T_3 + H_3;

% Sum up the rotor forces in the z-direction from each vector to get the
% total body force in the z-direction
B_Fr = B_Fr_0 + B_Fr_1 + B_Fr_2 + B_Fr_3;

% Define the in-plane drag and induced torque produced by each rotor
 B_Q_d0 = -1 * Kd * w_0 * w_0 * gamma_omega_03;
 B_Q_d1 = -1 * Kd * w_1 * w_1 * gamma_omega_12;
 B_Q_d2 = -1 * Kd * w_2 * w_2 * gamma_omega_12;
 B_Q_d3 = -1 * Kd * w_3 * w_3 * gamma_omega_03;

% Sum up the total in-plane drag and induced torque to get the total
% in-plane drag and induced torque on the body
B_Q_d = B_Q_d0 + B_Q_d1 + B_Q_d2 + B_Q_d3;

% Define the force lever arm torque created from the force produced by each
% rotor in the z-direction
B_Q_F0 = cross( rh_0, B_Fr_0 );
B_Q_F1 = cross( rh_1, B_Fr_1 );
B_Q_F2 = cross( rh_2, B_Fr_2 );
B_Q_F3 = cross( rh_3, B_Fr_3 );

B_Q_F = B_Q_F0 + B_Q_F1 + B_Q_F2 + B_Q_F3;

% Define the change in angular momentum torque produced by each rotor 
B_Q_L0 = -1 * Jreq * ( cross(B_omega, w_0 * gamma_omega_03) + w_0_dot * gamma_omega_03 );
B_Q_L1 = -1 * Jreq * ( cross(B_omega, w_1 * gamma_omega_12) + w_1_dot * gamma_omega_12 ); 
B_Q_L2 = -1 * Jreq * ( cross(B_omega, w_2 * gamma_omega_12) + w_2_dot * gamma_omega_12 ); 
B_Q_L3 = -1 * Jreq * ( cross(B_omega, w_3 * gamma_omega_03) + w_3_dot * gamma_omega_03 );

% Sum up the total change in angular momentum torque produced by each rotor
B_Q_L = B_Q_L0 + B_Q_L1 + B_Q_L2 + B_Q_L3;
    
% Define the total rotor system torque as the sum of the in-plane drag and
% induced torque, force lever arm torque, and change in angular momentum
% torques
B_Q = B_Q_d + B_Q_F + B_Q_L;

% Define the body forces in the z-direction from each vector to get the
% total body force in the z-direction
B_F = B_Fr + B_Fg; 

% Determine the dynamics of the system
M = [m * I , -m * r_oc_X; 
    zeros(3,3), J];

dynamics = M^-1*[B_F - m*cross(B_omega,B_vo) - m*cross(B_omega,cross(B_omega,r_oc)) ; ... 
          B_Q - cross(B_omega,J*B_omega) - cross(r_oc,B_F) ];

% Define the body frame angular velocities
B_vo_dot = dynamics(1:3);

% Define the body frame linear velocities
B_omega_dot = dynamics(4:6);

== matlab function test_model/Actuation/Aeb














 ==
function euler_rates = angular_body_earth_conversion(B_omega, euler_angles)

phi = euler_angles(1);
theta = euler_angles(2);

Aeb = [1,  sin(phi)*tan(theta), cos(phi)*tan(theta); ...
       0,      cos(phi)       ,        -sin(phi)   ; ...
       0,  sin(phi)/cos(theta), cos(phi)/cos(theta)];

   
euler_rates = Aeb * B_omega;

== matlab function test_model/Actuation/Lbe

















 ==
function [B_Fg, B_g]  = linear_earth_body_conversion(E_Fg, euler_angles, m)

phi = euler_angles(1);
theta = euler_angles(2);
psi = euler_angles(3);

Lbe = [             cos(theta)*cos(psi)              ,          cos(theta)*sin(psi)                  ,     -sin(theta)    ; ...
       sin(phi)*sin(theta)*cos(psi)-cos(phi)*sin(psi), sin(phi)*sin(theta)*sin(psi)+cos(phi)*cos(psi), sin(phi)*cos(theta); ...
       cos(phi)*sin(theta)*cos(psi)+sin(phi)*sin(psi), cos(phi)*sin(theta)*sin(psi)-sin(phi)*cos(psi), cos(phi)*cos(theta)];

B_Fg = Lbe * E_Fg;

B_g = B_Fg/m;

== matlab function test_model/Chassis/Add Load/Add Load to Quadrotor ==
function [m,J,r_oc] = add_load(m_0,J_0,r_oc_0,m_l,J_l,r_ol)
%#codegen
r_oc = (m_0*r_oc_0 + m_l*r_ol)/(m_0+m_l); 
m = m_0 + m_l; 
r_cl = -r_oc + r_ol; 
r_co = -r_oc; 
J = J_0 + J_l + m_0*(r_co'*r_co*eye(3) - r_co*r_co') + m_l*(r_cl'*r_cl*eye(3) - r_cl*r_cl'); 

end

== matlab function test_model/     Sensors   /IMU





/






 ==
function [accelReading,gyroReading] = idealIMU(B_vo_dot, B_vo, B_Omega, B_g, g, r_oc)
%#codegen

a = B_vo_dot + cross(B_Omega,B_vo); % body frame acceleration 

accelReading = (a - B_g)/g ; % accelerometer reading (ideal)

gyroReading = B_Omega ; % gyroscope reading (ideal) 

end

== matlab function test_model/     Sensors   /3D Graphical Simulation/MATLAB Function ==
function y = eigenaxis_ucart(u)


if abs(u(1))< 0.0001
    u(1) = 0.0001;
end

if abs(u(2))< 0.0001
    u(2) = 0.0001;
end

if abs(u(3))< 0.0001
    u(3) = 0.0001;
end

u = [ -u(1); -u(2); u(3) ];% [Pitch, Yaw, Roll] 

C11 = cos(u(2))*cos(u(3));
C12 = cos(u(2))*sin(u(3));
C13 = -sin(u(2));
C21 = sin(u(1))*sin(u(2))*cos(u(3))-cos(u(1))*sin(u(3));
C22 = sin(u(1))*sin(u(2))*sin(u(3))+cos(u(1))*cos(u(3));
C23 = sin(u(1))*cos(u(2));
C31 = cos(u(1))*sin(u(2))*cos(u(3))+sin(u(1))*sin(u(3));
C32 = cos(u(1))*sin(u(2))*sin(u(3))-sin(u(1))*cos(u(3));
C33 = cos(u(1))*cos(u(2));
    
theta = acos(0.5*(C11+C22+C33-1));

e = [C23-C32; C31-C13; C12-C21]/(2*sin(theta));
    
y = [e; theta];

== matlab function test_model/     Sensors   /Aeb









 ==
function euler_rates_IMU = angular_body_earth_conversion(gyro_reading, euler_angles_filtered)

phi = euler_angles_filtered(1);
theta = euler_angles_filtered(2);

Aeb = [1, sin(phi)*tan(theta), cos(phi)*tan(theta); ...
       0,     cos(phi)       ,        -sin(phi)   ; ...
       0,  sin(phi)/cos(theta), cos(phi)/cos(theta)];

   
euler_rates_IMU = Aeb * gyro_reading;

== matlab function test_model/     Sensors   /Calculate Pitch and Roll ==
function [accel_pitch, accel_roll] = getPitchAndRoll(accel_reading)

x_accel = accel_reading(1);
y_accel = accel_reading(2);
z_accel = accel_reading(3);

accel_pitch = atan(x_accel/sqrt(y_accel^2 + z_accel^2));
accel_roll = atan( -y_accel/( sqrt(z_accel^2 + x_accel^2))  );

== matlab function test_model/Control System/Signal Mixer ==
function P  = signal_mixer(height_controlled, y_controlled, x_controlled, yaw_controlled)

controller_outputs = [ height_controlled; x_controlled; y_controlled; yaw_controlled ];
signal_mixer = [ 1, -1, -1, -1; ... 
                 1,  1, -1,  1; ...
                 1, -1,  1,  1; ...
                 1,  1,  1, -1 ];
             
P = signal_mixer * controller_outputs;

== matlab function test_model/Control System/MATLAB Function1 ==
function [z_corr, y_cor, x_corr, yaw_corr, pid_y_out, pid_roll_out] = c_controller(set_x, set_y, set_z, set_yaw, ...
    cur_x, cur_y, cur_z, ...
    cur_phi, cur_theta, cur_psi, ...
    cur_phi_d, cur_theta_d, cur_psi_d, vrpn_id, Tc)

out_z = -1;
out_y = -1;
out_x = -1;
out_yaw = -1;
c_pid_y = -1;
c_pid_roll = -1;

coder.ceval('c_controller', vrpn_id, Tc, set_x, set_y, set_z, set_yaw, ...
                    cur_x, cur_y, cur_z, ...
                    cur_phi, cur_theta, cur_psi, ...
                    cur_phi_d, cur_theta_d, cur_psi_d, ...
                    coder.wref(out_z), coder.wref(out_y), coder.wref(out_x), coder.wref(out_yaw), ...
                    coder.wref(c_pid_y), coder.wref(c_pid_roll));

z_corr = out_z;
y_cor = out_y;
x_corr = out_x;
pid_y_out = c_pid_y;
pid_roll_out = c_pid_roll;
yaw_corr = out_yaw;

== matlab function test_model/     Sensors   /Aeb_c









1 ==
function euler_rates_IMU = angular_body_earth_conversion(gyro_reading, euler_angles_filtered)

phi = euler_angles_filtered(1);
theta = euler_angles_filtered(2);
psi = NaN;

phi_dot = -1;
theta_dot = -1;
psi_dot = -1;

p = gyro_reading(1);
q = gyro_reading(2);
r = gyro_reading(3);

coder.ceval( 'aeb_mat', p, q, r, phi, theta, psi, coder.wref(phi_dot), ...
    coder.wref(theta_dot), coder.wref(psi_dot) );

   
euler_rates_IMU = [phi_dot; theta_dot; psi_dot];

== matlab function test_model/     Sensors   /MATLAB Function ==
function euler_angles_IMU  = complimentaryFilterC(accel_pitch, accel_roll, euler_rates_gyro)

euler_x = euler_rates_gyro(1);
euler_y = euler_rates_gyro(2);

filtered_pitch = -1;
filtered_roll = -1;

coder.ceval('compl_filter', accel_pitch, accel_roll, euler_x, euler_y, ...
            coder.wref(filtered_pitch), coder.wref(filtered_roll));

euler_angles_IMU = [filtered_roll; filtered_pitch];

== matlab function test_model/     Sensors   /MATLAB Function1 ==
function [accel_pitch, accel_roll]  = angle_IMU_C(accel_reading)

accel_x = accel_reading(1);
accel_y = accel_reading(2);
accel_z = accel_reading(3);

calculated_pitch = -1;
calculated_roll = -1;

coder.ceval('angle_accel', accel_x, accel_y, accel_z, coder.wref(calculated_pitch), coder.wref(calculated_roll));

accel_pitch = calculated_pitch;
accel_roll = calculated_roll;

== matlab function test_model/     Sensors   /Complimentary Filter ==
function euler_angles_IMU   = complimentaryFilter(accel_pitch, accel_roll, euler_rates_gyro, prev_euler_angles)

k_gyro = 0.99; 
k_accel = 1-k_gyro; 

Ts = 0.005; % 5 milliseconds

prev_phi = prev_euler_angles(1);
prev_theta = prev_euler_angles(2);

prev_phi_dot = euler_rates_gyro(1);
prev_theta_dot = euler_rates_gyro(2);

integrated_phi_gyro = Ts * prev_phi_dot + prev_phi;
integrated_theta_gyro = Ts * prev_theta_dot + prev_theta;

phi = k_gyro * integrated_phi_gyro + k_accel * accel_roll;
theta = k_gyro * integrated_theta_gyro + k_accel * accel_pitch;

euler_angles_IMU = [phi; theta];

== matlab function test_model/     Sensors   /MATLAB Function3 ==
function [eulerAngles, integralFeedback, quaternions] = ...
    mahonyFilter(accelReadings, gyroReadings, quaternions_prev, ...
    integralFeedback_prev, Tq, Kp_mahony, Ki_mahony)
%     mahonyFilter(accelReadings, gyroReadings, eulerAngles_prev, ...
%     integralFeedback_prev, Tq, Kp_mahony, Ki_mahony)
    
    
    %Save quadcopter loop time as dt
    dt = Tq;

    %Pull accelerometer readings and negate them to compare
    accel_x = accelReadings(1);
    accel_y = accelReadings(2);
    accel_z = accelReadings(3);
    
    %Negate the accelerometer values to compare with direction of the
    %gravity vector
    accel_x = (-1) * accel_x;
    accel_y = (-1) * accel_y;
    accel_z = (-1) * accel_z;

    %Pull gyroscope readings
    gyro_x = gyroReadings(1);
    gyro_y = gyroReadings(2);
    gyro_z = gyroReadings(3);

    %Pull previous Euler angles
%     roll_prev = eulerAngles_prev(1);
%     pitch_prev = eulerAngles_prev(2);
%     yaw_prev = eulerAngles_prev(3);
    
    %Pull previous integral feedback terms
    integralFeedback_x_prev = integralFeedback_prev(1);
    integralFeedback_y_prev = integralFeedback_prev(2);
    integralFeedback_z_prev = integralFeedback_prev(3);

    %Calculate half cosines and sines for the quaternion elements
%     cosHalfRoll = cos( 0.5 * roll_prev );
%     sinHalfRoll = sin( 0.5 * roll_prev );
%     cosHalfPitch = cos( 0.5 * pitch_prev );
%     sinHalfPitch = sin( 0.5 * pitch_prev );
%     cosHalfYaw = cos( 0.5 * yaw_prev );
%     sinHalfYaw = sin( 0.5 * yaw_prev );

    %Calculate the quaternion elements
%     q0 = cosHalfRoll * cosHalfPitch * cosHalfYaw + ...
%         sinHalfRoll * sinHalfPitch * sinHalfYaw;
% 
%     q1 = sinHalfRoll * cosHalfPitch * cosHalfYaw - ...
%         cosHalfRoll * sinHalfPitch * sinHalfYaw;
% 
%     q2 = cosHalfRoll * sinHalfPitch * cosHalfYaw + ...
%         sinHalfRoll * cosHalfPitch * sinHalfYaw;
% 
%     q3 = (-1) * sinHalfRoll * sinHalfPitch * cosHalfYaw + ...
%         cosHalfRoll * cosHalfPitch * sinHalfYaw;

    %Pull the quaternion values
    q0 = quaternions_prev(1);
    q1 = quaternions_prev(2);
    q2 = quaternions_prev(3);
    q3 = quaternions_prev(4);


    %Calculate the rate of change of the quaternion from the gyroscope
%     q0_dot = 0.5 * ( (-1)*(q1 * gyro_x) - (q2 * gyro_y) - (q3 * gyro_z) );
%     q1_dot = 0.5 * ( (q0 * gyro_x) + (q2 * gryo_z) - (q3 * gyro_y) );
%     q2_dot = 0.5 * ( (q0 * gyro_y) - (q1 * gyro_z) + (q3 * gyro_x) );
%     q3_dot = 0.5 * ( (q0 * gyro_z) + (q1 * gyro_y) - (q2 * gyro_x) );

    %Define initial values for the corrected gyroscope values
    gyro_x_corrected = gyro_x;
    gyro_y_corrected = gyro_y;
    gyro_z_corrected = gyro_z;
    
    %Define initial values for the corrected integral feedback values
    integralFeedback_x = integralFeedback_x_prev;
    integralFeedback_y = integralFeedback_y_prev;
    integralFeedback_z = integralFeedback_z_prev;

    %Only compute the feedback if the accelerometer measurements are valid
    %This prevents NaN values when normalizing the accelerometer measurements
    if( accel_x ~= 0 && accel_y ~= 0  && accel_z ~= 0 )

       %Check... maybe we don't need to do this normalization...
       %Ideally our accelerometer readings should have a magnitude of 1, but
       %this is usually not the case with data we have collected
       accel_mag = ( (accel_x ^ 2) + (accel_y ^ 2) + (accel_z ^ 2) ) ^ 0.5;
       accel_x = accel_x / accel_mag;
       accel_y = accel_y / accel_mag;
       accel_z = accel_z / accel_mag;

       %Estimate direction of gravity
       vx = 2 * ( (q1 * q3) - (q0 * q2) );
       vy = 2 * ( (q0 * q1) + (q2 * q3) );
       vz = (2 * q0 * q0) - (q3 * q3);
       
       %Error is the sum of the cross product between the estimated and
       %measured direction of gravity
       ex = (accel_y * vz) - (accel_z * vy);
       ey = (accel_z * vx) - (accel_x * vz);
       ez = (accel_x * vy) - (accel_y * vx);
       
       %Compute and apply the proportional feedback
       gyro_x_corrected = gyro_x + (Kp_mahony * ex);
       gyro_y_corrected = gyro_y + (Kp_mahony * ey);
       gyro_z_corrected = gyro_z + (Kp_mahony * ez);

       %Compute and apply the integral feedback, if it is enabled
       if ( Ki_mahony > 0 )
           
           %Integrate digitally based on sample time and scale by Ki, and
           %accumulate the integral term by adding this to the previous
           %feedback term
           integralFeedback_x = (Ki_mahony * ex * dt) + ...
               integralFeedback_x_prev;
           integralFeedback_y = (Ki_mahony * ey * dt) + ...
               integralFeedback_y_prev;
           integralFeedback_z = (Ki_mahony * ez * dt) + ...
               integralFeedback_z_prev;
           
           %Correct the gyroscope values using the new integral feedback
           gyro_x_corrected = gyro_x_corrected + integralFeedback_x;
           gyro_y_corrected = gyro_y_corrected + integralFeedback_y;
           gyro_z_corrected = gyro_z_corrected + integralFeedback_z;
           
       else
           
           %Otherwise, reset the integral terms to zero to prevent windup
           integralFeedback_x = 0;
           integralFeedback_y = 0;
           integralFeedback_z = 0;
           
       end %if ( Ki_mahoney > 0 )

    end %if ( accel_x ~= 0 && accel_y ~= 0 && accel_z ~= 0 )

    %Integrate the rate of change of the quaternion
    %First, pre-multiply the common factors to the gyro reading values
    gyro_x_corrected = gyro_x_corrected * (0.5 * dt);
    gyro_y_corrected = gyro_y_corrected * (0.5 * dt);
    gyro_z_corrected = gyro_z_corrected * (0.5 * dt);
    
    %Now, create temporary variales for the first three quaternion values
    qa = q0;
    qb = q1;
    qc = q2;
    
    %Now perform calculation to integrate the rate of the quaternion
    q0 = q0 - (qb * gyro_x_corrected) - (qc * gyro_y_corrected) - ...
        (q3 * gyro_z_corrected);
    q1 = q1 + (qa * gyro_x_corrected) + (qc * gyro_z_corrected) - ...
        (q3 * gyro_y_corrected);
    q2 = q2 + (qa * gyro_y_corrected) - (qb * gyro_z_corrected) + ...
        (q3 * gyro_x_corrected);
    q3 = q3 + (qa * gyro_z_corrected) + (qb * gyro_y_corrected) - ...
        (qc * gyro_x_corrected);
    
    %Normalize quaternion
    quaternion_mag = ( (q0 * q0) + (q1 * q1) + (q2 * q2) + (q3 * q3) ) ^ 0.5;
    q0 = q0 / quaternion_mag;
    q1 = q1 / quaternion_mag;
    q2 = q2 / quaternion_mag;
    q3 = q3 / quaternion_mag;
    
    %Estimate the gravity direction from the quaternion values
    grav_x = 2 * ( (q1 * q3) - (q0 * q2) );
    grav_y = 2 * ( (q0 * q1) + (q2 * q3) );
    grav_z = (q0 * q0) - (q1 * q1) - (q2 * q2) + (q3 * q3);
    
    %Limit the gravity vector in x-direction to maintain a magnitude of 1
%     grav_x = min( grav_x , 1 );
%     grav_x = max( grav_x , -1 );

    %Normalize the gravity vector
    grav_mag = sqrt( ( grav_x * grav_x ) + ( grav_y * grav_y ) + ...
        ( grav_z * grav_z ) );
    grav_x = grav_x / grav_mag;
    grav_y = grav_y / grav_mag;
    grav_z = grav_z / grav_mag;
    
    %Calculate the pitch, roll, and yaw
    yaw = atan2( 2 * ( (q0 * q3) + (q1 * q2) ) , ...
        (q0 * q0) + (q1 * q1) - (q2 * q2) - (q3 * q3) );
    pitch = asin( (-1) * grav_x );
    roll = atan2( grav_y , grav_z );
    
    %Create a vector of current integral feedback terms to output
    integralFeedback = [ integralFeedback_x ; ...
        integralFeedback_y ; integralFeedback_z ];
    
    %Create a vector of the corrected gyroscope terms
    %gyroReadings_corrected = [ gyro_x_corrected ; ...
    %    gyro_y_corrected ; gyro_z_corrected ];
    
    %Create a vector of the newly calculated quaternion values
    quaternions = [ q0 ; q1 ; q2 ; q3 ];
    
    %Create a vector of the calculated Euler angles
    eulerAngles = [ roll ;  pitch ; yaw ];
    
end %function

== matlab function test_model/Chassis/Body Frame 
Angular Velocity 
to Euler Rates ==
function dot_Theta = pqr2euler(Omega_B,Theta)
%#codegen

phi = Theta(1); 
theta = Theta(2); 
%psi = Theta(3); 

A_BE = [ 1 sin(phi)*tan(theta) cos(phi)*tan(theta); 
         0      cos(phi)            -sin(phi)     ; 
         0 sin(phi)/cos(theta) cos(phi)/cos(theta) ];
     
dot_Theta = A_BE*Omega_B; 

end
